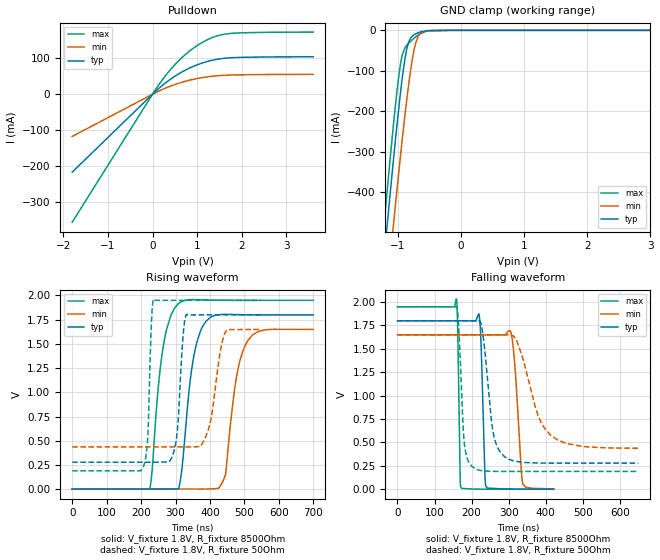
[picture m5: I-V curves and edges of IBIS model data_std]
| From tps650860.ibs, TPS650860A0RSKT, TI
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|   data_std Model
[Model]   data_std
Model_type   I/O_open_drain
Polarity   Inverting
Vinl = 0.4
Vinh = 1.2
Vmeas = 0.9
Vref = 1.8
Cref = 50pF
Rref = 8500
|   typ   min   max
|   (nom PVT)   (fast PVT)   (slow PVT)
C_comp   1.676e-12   1.451e-12   1.832e-12
| Where nom  PVT is Nominal Process, 1.8V, 27C
|   Fast PVT is Strong Process,  1.95V, -40C
|   Slow PVT is Weak Process,   1.65V, 125C
[Voltage Range]   1.8   1.65   1.95
|Junction Temperature
[Temperature Range]   27   125   -40
[Pullup Reference]   1.8   1.65   1.95
[Pulldown Reference]   0   0   0
[Power Clamp Reference]   1.8   1.65   1.95
[GND Clamp Reference]   0   0   0
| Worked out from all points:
|   slope of the pulldown table from 0 to 0.27 V, typ, clamps not added: 9.17 ohm
|   GND clamp passes 1 mA (typ) near -0.54 V on its own axis
|   falling waveform, V_fixture 1.8V, R_fixture 8500Ohm: 20-80 % time 7.89ns typ, 15.2ns min, 4.9ns max; typ from 1.8 V to 0.002 V
|   rising waveform, V_fixture 1.8V, R_fixture 8500Ohm: 20-80 % time 34ns typ, 36ns min, 32.7ns max; typ from 0.002 V to 1.8 V
|   falling waveform, V_fixture 1.8V, R_fixture 50Ohm: 20-80 % time 24.1ns typ, 55.2ns min, 12.3ns max; typ from 1.8 V to 0.28 V
|   rising waveform, V_fixture 1.8V, R_fixture 50Ohm: 20-80 % time 15.5ns typ, 29.3ns min, 9.02ns max; typ from 0.28 V to 1.8 V
[Pulldown]
|   Voltage   I(typ)   I(min)   I(max)
-1.8V     -217.2mA   -117.7mA   -356.6mA
117mV     13.52mA    7.322mA    22.21mA
321.9mV   34.46mA    18.63mA    56.63mA
467.8mV   47.38mA    25.58mA    77.92mA
684mV     63.67mA    34.26mA    104.9mA
826.2mV   72.65mA    38.98mA    120mA
1.081V    85.55mA    45.61mA    141.9mA
1.263V    92.42mA    49mA       153.8mA
1.398V    96.23mA    50.82mA    160.5mA
1.642V    100.5mA    52.87mA    167.8mA
1.981V    102.8mA    54.13mA    171.1mA
3.6V      104.4mA    55.46mA    173.2mA
[GND Clamp]
|   Voltage   I(typ)   I(min)   I(max)
-1.8V     -1.585A    -1.712A    -1.529A
-1.417V   -903.9mA   -1.052A    -830.1mA
-1.201V   -532.4mA   -690.5mA   -448.4mA
-1.17V    -480.2mA   -639.5mA   -395mA
-1.076V   -327.4mA   -488.9mA   -240.6mA
-959.6mV  -153.1mA   -309.5mA   -82.58mA
-887.4mV  -67.95mA   -206.8mA   -42.91mA
-828mV    -27.88mA   -130.5mA   -31.56mA
-722.6mV  -8.948mA   -32.89mA   -16.64mA
-648.3mV  -4.138mA   -7.502mA   -8.538mA
-516.9mV  -657.9uA   -778.2uA   -1.114mA
3.6V      0A         0A         0A
[POWER Clamp]
|   Voltage   I(typ)   I(min)   I(max)
-1.8V     0A         0A         0A
0V        0A         0A         0A
3.6V      0A         0A         0A
[Ramp]
R_load = 8500
|   typ   min   max
dV/dt_r   1.07894/3.39515e-08   0.988027/3.59962e-08   1.1693/3.26022e-08
dV/dt_f   1.07894/7.85826e-09   0.988028/1.51363e-08   1.1693/4.88369e-09
[Falling Waveform]
V_fixture = 1.8V
V_fixture_min = 1.65V
V_fixture_max = 1.95V
R_fixture = 8500Ohm
|   Time   V(typ)   V(min)   V(max)
0s        1.8V       1.65V      1.95V
159.4ns   1.8V       1.65V      2.032V
162.1ns   1.8V       1.65V      1.761V
170.4ns   1.8V       1.65V      26.72mV
219.3ns   1.874V     1.65V      1.359mV
225.1ns   1.593V     1.65V      1.297mV
238.2ns   34.84mV    1.65V      1.213mV
305ns     2.11mV     1.69V      1.157mV
337.1ns   1.843mV    77.14mV    1.157mV
421.4ns   1.755mV    4.221mV    1.157mV
[Rising Waveform]
V_fixture = 1.8V
V_fixture_min = 1.65V
V_fixture_max = 1.95V
R_fixture = 8500Ohm
|   Time   V(typ)   V(min)   V(max)
0s        1.754mV    2.968mV    1.157mV
225.5ns   1.754mV    2.968mV    2.734mV
264.5ns   1.754mV    2.968mV    1.476V
309.3ns   5.027mV    2.968mV    1.918V
351.4ns   1.34V      2.968mV    1.957V
389.1ns   1.735V     3.139mV    1.953V
445.3ns   1.805V     152.6mV    1.95V
477.1ns   1.803V     1.157V     1.95V
508.9ns   1.801V     1.529V     1.95V
699.8ns   1.8V       1.65V      1.95V
[Falling Waveform]
V_fixture = 1.8V
V_fixture_min = 1.65V
V_fixture_max = 1.95V
R_fixture = 50Ohm
|   Time   V(typ)   V(min)   V(max)
0s        1.8V       1.65V      1.95V
160ns     1.8V       1.65V      1.95V
180.8ns   1.8V       1.65V      479.6mV
210.7ns   1.8V       1.65V      217.2mV
228.5ns   1.711V     1.65V      198.8mV
259.7ns   576.9mV    1.65V      191.6mV
288.5ns   349.9mV    1.65V      190.6mV
322.9ns   295.6mV    1.574V     190.5mV
414.2ns   279.7mV    574.7mV    190.5mV
649.8ns   279.5mV    438.2mV    190.5mV
[Rising Waveform]
V_fixture = 1.8V
V_fixture_min = 1.65V
V_fixture_max = 1.95V
R_fixture = 50Ohm
|   Time   V(typ)   V(min)   V(max)
0s        279.5mV    438.2mV    190.5mV
206.3ns   279.5mV    438.2mV    228.9mV
219.7ns   279.5mV    438.2mV    543.5mV
230.2ns   279.5mV    438.2mV    1.727V
237.8ns   279.5mV    438.2mV    1.963V
299.3ns   449.5mV    438.2mV    1.95V
332.4ns   1.807V     438.2mV    1.95V
394.7ns   1.8V       607.5mV    1.95V
446.2ns   1.8V       1.631V     1.95V
549.8ns   1.8V       1.65V      1.95V
